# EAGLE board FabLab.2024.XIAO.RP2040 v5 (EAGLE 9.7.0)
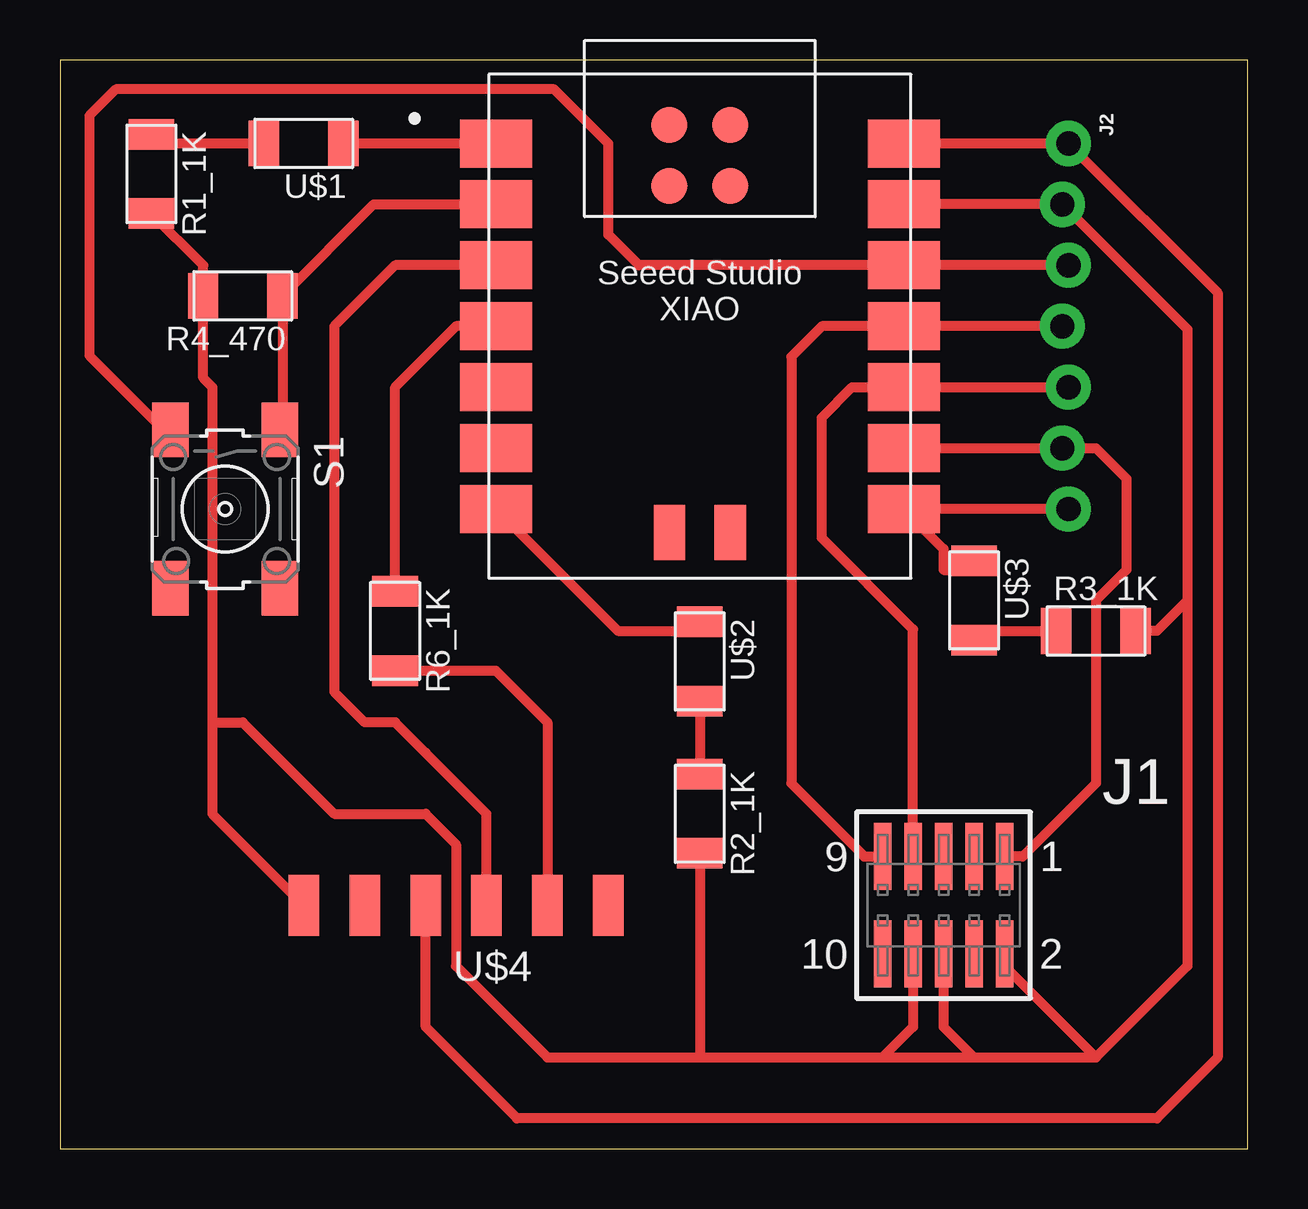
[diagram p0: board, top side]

Size 49.51 x 45.39 mm. Coordinates in mm from the lower left corner, seen from the top.
Outline: 0,0 49.51,0 49.51,45.39 0,45.39 0,0
Copper layers (1*16): Top 0.035mm / dielectric 1.5mm / Bottom 0.035mm
Design rules "default": minimum track width 6mil, minimum drill 0.35mm, track to track 6mil, track to pad 6mil, pad to pad 6mil, via to via 6mil, smd to smd 6mil, copper to edge 40mil, drill to drill 6mil, minimum pad ring 10mil, minimum via ring 8mil, stop-mask expansion 4mil, vias tented up to drill 0mil, thermal gap 10mil

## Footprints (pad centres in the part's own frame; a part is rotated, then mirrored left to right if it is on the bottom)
SAMTEC-FTS-105-01-X-DV = smd 0.74 x 2.79: 1 -2.54,-2.032; 2 -2.54,2.032; 3 -1.27,-2.032; 4 -1.27,2.032; 5 0,-2.032; 6 0,2.032; 7 1.27,-2.032; 8 1.27,2.032; 9 2.54,-2.032; 10 2.54,2.032
1X07_LOCK_NO_SILK = drill 1.016 pad 1.88: 1 0,0.127; 2 2.54,-0.127; 3 5.08,0.127; 4 7.62,-0.127; 5 10.16,0.127; 6 12.7,-0.127; 7 15.24,0.127
R1206FAB = smd 1.27 x 1.905: 1 -1.651,0; 2 1.651,0
6MM_SWITCH = smd 2.286 x 1.524: 1 -3.302,2.286; 2 3.302,2.286; 3 -3.302,-2.286; 4 3.302,-2.286
XIAO-SAMD21/RP2040-MODULE14P-2.54-21X17.8MM = smd 3 x 2: 1 -8.5,7.62; 2 -8.5,5.08; 3 -8.5,2.54; 4 -8.5,0; 5 -8.5,-2.54; 6 -8.5,-5.08; 7 -8.5,-7.62; 8 8.5,-7.62; 9 8.5,-5.08; 10 8.5,-2.54; 11 8.5,0; 12 8.5,2.54; 13 8.5,5.08; 14 8.5,7.62 | smd 1.5 x 1.5: 15 -1.27,8.39; 16 1.27,8.39; 17 -1.27,5.85; 18 1.27,5.85 | smd 1.3 x 2.3: 19 -1.27,-8.6; 20 1.27,-8.6
LED1206FAB = smd 1.27 x 1.905: 1 -1.651,0; 2 1.651,0
1X06SMD = smd 2.54 x 1.27: 1 0,6.35; 2 0,3.81; 3 0,1.27; 4 0,-1.27; 5 0,-3.81; 6 0,-6.35

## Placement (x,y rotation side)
J1  SAMTEC-FTS-105-01-X-DVJ  [SAMTEC-FTS-105-01-X-DV]  36.83,10.16 180 top
J2  [1X07_LOCK_NO_SILK]  41.91,41.91 270 top
R1_1K  [R1206FAB]  3.81,40.64 270 top
R2_1K  [R1206FAB]  26.67,13.97 270 top
R3_1K  [R1206FAB]  43.18,21.59 0 top
R4_470  [R1206FAB]  7.62,35.56 180 top
R6_1K  [R1206FAB]  13.97,21.59 270 top
S1  [6MM_SWITCH]  6.88,26.67 270 top
U1  XIAO-RP2040  [XIAO-SAMD21/RP2040-MODULE14P-2.54-21X17.8MM]  26.67,34.29 0 top
U$1  LEDFAB1206  [LED1206FAB]  10.16,41.91 180 top
U$2  LEDFAB1206  [LED1206FAB]  26.67,20.32 270 top
U$3  LEDFAB1206  [LED1206FAB]  38.1,22.86 270 top
U$4  CONN_06_FTDI-SMD-HEADER  [1X06SMD]  16.51,10.16 90 top

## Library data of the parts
J1 = SAMTEC-FTS-105-01-X-DV; AVAILABILITY: In Stock; CHECK_PRICES: https://www.snapeda.com/parts/FTS-105-01-S-DV/Samtec/view-part/?ref=eda; DESCRIPTION: Conn Unshrouded Header HDR 10 POS 1.27mm Solder ST SMD Tube; MF: Samtec; MP: FTS-105-01-S-DV; PACKAGE: None; PRICE: None; PURCHASE-URL: https://www.snapeda.com/api/url_track_click_mouser/?unipart_id=3340737&manufacturer=Samtec&part_name=FTS-105-01-S-DV&search_term=conn header smd 10pos 1.27mm; SNAPEDA_LINK: https://www.snapeda.com/parts/FTS-105-01-S-DV/Samtec/view-part/?ref=snap
J2 = SparkFun-Connectors
R1_1K R2_1K R3_1K R4_470 R6_1K S1 U$1-U$4 = fab
U1 = Seeed Studio XIAO Series

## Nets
BUTTON: R4_470.1 S1.1 U1.2
HELLO_LED: U1.1 U$1.1
N$1: R2_1K.1 U$2.2
N$2: R3_1K.1 U$3.2
N$3: R1_1K.1 U$1.2
N$4: R6_1K.1 U1.4
N$14: S1.4
NC: J1.3
PWR_3V3: J2.3 S1.3 U1.12
PWR_5V: J2.1 U1.14 U$4.3
PWR_GND: J1.2 J1.6 J1.8 J2.2 R1_1K.2 R2_1K.2 R3_1K.2 R4_470.2 U1.13 U$4.1
SWAD_TARG_VCC: J1.10
SWD_KEY: J1.4
SWD_LED: J2.7 U1.8 U$3.1
SWD_RST: J1.1 J2.6 U1.9
SWD_SWCLK: J1.7 J2.5 U1.10
SWD_SWDIO: J1.9 J2.4 U1.11
SWD_SWO: J1.5
UART_LED: U1.7 U$2.1
UART_RX: R6_1K.2 U$4.5
UART_TX: U1.3 U$4.4

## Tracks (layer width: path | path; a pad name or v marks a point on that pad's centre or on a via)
BUTTON
  Top 0.406: U1.2 13.08,39.37 R4_470.1 9.27,30.07 S1.1
HELLO_LED
  Top 0.406: U1.1 U$1.1
N$1
  Top 0.406: U$2.2 R2_1K.1
N$2
  Top 0.406: U$3.2 38.48,21.59 R3_1K.1
N$3
  Top 0.406: U$1.2 4.19,41.91 R1_1K.1
N$4
  Top 0.406: R6_1K.1 13.97,31.75 16.51,34.29 U1.4
PWR_3V3
  Top 0.406: J2.3 U1.12 24.13,36.83 22.86,38.1 22.86,41.91 20.6,44.17 2.33,44.17 1.22,43.06 1.22,33.07 3.17,31.11 3.81,30.48 4.32,29.97 S1.3
PWR_5V
  Top 0.406: U1.14 J2.1 48.26,35.69 48.26,3.81 45.72,1.27 19.05,1.27 15.24,5.08 U$4.3
PWR_GND
  Top 0.406: U1.13 J2.2 46.99,34.16 46.99,22.86 | R1_1K.2 5.97,36.83 R4_470.2 5.97,32.13 6.35,31.75 6.35,17.78 | 6.35,17.78 6.35,13.97 U$4.1 | R2_1K.2 26.67,3.81 | 46.99,22.86 45.72,21.59 R3_1K.2 | 46.99,22.86 46.99,7.62 43.18,3.81 | 6.35,17.78 7.62,17.78 11.43,13.97 15.24,13.97 16.51,12.7 16.51,7.62 20.32,3.81 26.67,3.81 | 26.67,3.81 34.29,3.81 | 34.29,3.81 38.1,3.81 | 38.1,3.81 43.18,3.81 | J1.2 39.37,7.62 43.18,3.81 | J1.6 36.83,5.08 38.1,3.81 | J1.8 35.56,5.08 34.29,3.81
SWD_LED
  Top 0.406: J2.7 U1.8 36.83,25.01 36.83,24.13 37.72,24.13 U$3.1
SWD_RST
  Top 0.406: U1.9 J2.6 43.18,29.21 44.45,27.94 44.45,24.13 43.18,22.86 43.18,15.24 40.13,12.19 J1.1 39.37,12.7
SWD_SWCLK
  Top 0.406: J2.5 U1.10 33.02,31.75 31.75,30.48 31.75,25.47 35.56,21.66 J1.7
SWD_SWDIO
  Top 0.406: J2.4 U1.11 31.75,34.29 30.48,33.02 30.48,15.24 33.53,12.19 J1.9
UART_LED
  Top 0.406: U$2.1 26.29,21.59 23.25,21.59 U1.7
UART_RX
  Top 0.406: R6_1K.2 18.16,19.94 20.32,17.78 U$4.5
UART_TX
  Top 0.406: U$4.4 17.78,13.97 15.24,16.51 13.97,17.78 12.7,17.78 11.43,19.05 11.43,34.29 13.97,36.83 U1.3 19.05,36.83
